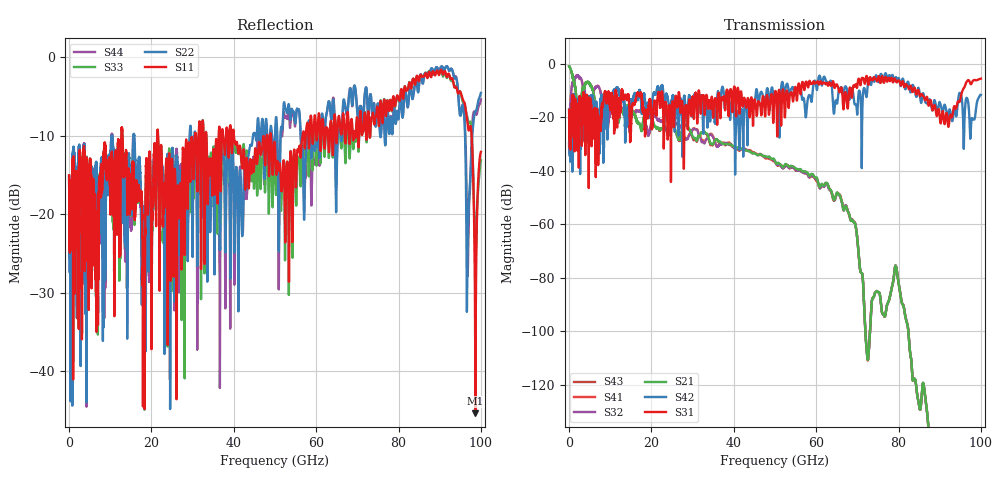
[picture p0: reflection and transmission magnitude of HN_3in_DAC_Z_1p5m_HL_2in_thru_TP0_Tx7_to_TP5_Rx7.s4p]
# GHz S RI R 45
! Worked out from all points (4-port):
!   4000 points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, 25 MHz to 100 GHz, reference 45 ohm
!   strongest paths, dB at 25 MHz, 25.02 GHz, 50.02 GHz, 75.03 GHz, 100 GHz:
!     S31: -17.1, -15.0, -10.4, -5.1, -5.5
!     S42: -17.1, -12.8, -11.9, -6.5, -11.5
!     S21: -0.8, -22.6, -36.3, -85.4, -
!     S32: -29.7, -23.3, -36.4, -85.4, -
!     S41: -29.7, -23.3, -36.5, -85.4, -
!     S43: -0.8, -23.0, -36.6, -85.4, -
!   lowest |S11| = -45.3 dB at 98.67 GHz (marker M1), VSWR 1.01, Z = 45.5 - j0.0597 ohm
!   |S11| at or under -10 dB: start of sweep to 12.69 GHz; 12.99 GHz to 21.41 GHz (8.42 GHz wide, 48.9 % of centre); 21.64 GHz to 30.58 GHz (8.94 GHz wide, 34.2 % of centre)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
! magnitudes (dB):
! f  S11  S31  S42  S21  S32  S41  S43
! 25 MHz  -15.0  -17.1  -17.1  -0.8  -29.7  -29.7  -0.8
! 2.2 GHz  -19.3  -21.1  -14.1  -25.3  -4.5  -4.5  -25.0
! 57.45 GHz  -10.2  -6.9  -19.8  -40.3  -40.6  -40.6  -40.9
! 71.72 GHz  -7.3  -7.0  -9.1  -93.0  -93.0  -92.9  -92.8
! 90.67 GHz  -2.1  -17.7  -18.0  -144.0  -143.8  -144.2  -144.0
! 98.67 GHz  -45.3  -6.0  -18.7  -  -  -  -
! 100 GHz  -12.1  -5.5  -11.5  -  -  -  -
